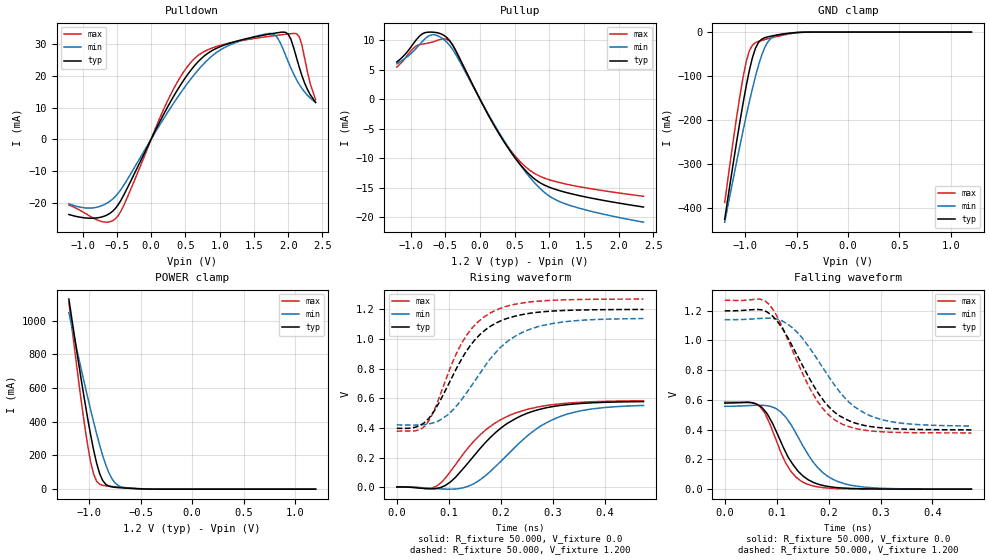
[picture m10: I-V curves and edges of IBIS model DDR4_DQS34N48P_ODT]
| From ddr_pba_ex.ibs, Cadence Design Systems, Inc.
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|   Model DDR4_DQS34N48P_ODT
[Model]   DDR4_DQS34N48P_ODT
Model_type I/O
Polarity   Non-Inverting
Enable   Active-High
Vinl =  0.823V
Vinh =  0.887V
C_comp   1.693pF   1.693pF   1.716pF
C_comp_pullup   0.525pF   0.576pF   0.518pF
C_comp_pulldown   1.168pF   1.117pF   1.198pF
[Model Spec]
Vinh   0.887V   NA   NA
Vinl   0.823V   NA   NA
Vmeas   0.840V   NA   NA
[Add Submodel]
|  Submodel_name   Mode
DDR4_DQS_ODT60   Non-Driving
[Temperature Range]   27.000   0.125k   -40.000
[Voltage Range]   1.200V   1.140V   1.270V
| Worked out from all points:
|   slope of the pulldown table from 0 to 0.18 V, typ, clamps not added: 23.3 ohm
|   slope of the pullup table from 0 to 0.18 V, typ, clamps not added: 45.9 ohm
|   GND clamp passes 1 mA (typ) near -0.50 V on its own axis
|   POWER clamp passes 1 mA (typ) near -0.46 V on its own axis
|   rising waveform, R_fixture 50.000, V_fixture 0.0: 20-80 % time 103ps typ, 110ps min, 100ps max; typ from 0.002 V to 0.578 V
|   rising waveform, R_fixture 50.000, V_fixture 1.200: 20-80 % time 83.6ps typ, 98.4ps min, 73ps max; typ from 0.397 V to 1.2 V
|   falling waveform, R_fixture 50.000, V_fixture 0.0: 20-80 % time 53.7ps typ, 63.6ps min, 45.1ps max; typ from 0.579 V to 0 V
|   falling waveform, R_fixture 50.000, V_fixture 1.200: 20-80 % time 81ps typ, 91.3ps min, 75.1ps max; typ from 1.2 V to 0.399 V
[Pulldown]
|Voltage   I(typ)   I(min)   I(max)
-1.2V     -23.72mA   -20.38mA   -20.68mA
-840mV    -24.88mA   -21.61mA   -24.88mA
-520mV    -21.78mA   -18mA      -25.05mA
400mV     16.1mA     13.66mA    18.67mA
640mV     23.35mA    20.64mA    25.58mA
960mV     28.73mA    27.44mA    29.28mA
1.76V     33.27mA    33.33mA    32.54mA
1.84V     33.56mA    32.14mA    32.76mA
2V        33.13mA    24.48mA    33.18mA
2.12V     25.82mA    18.86mA    33.28mA
2.2V      20.09mA    16.05mA    29.74mA
2.4V      11.64mA    11.56mA    12.48mA
[Pullup]
|Voltage   I(typ)   I(min)   I(max)
-1.2V     6.276mA    5.968mA    5.424mA
-960mV    9.395mA    8.108mA    8.597mA
-840mV    10.98mA    9.634mA    9.283mA
-720mV    11.33mA    10.8mA     9.54mA
-560mV    11.02mA    10.4mA     10.13mA
-400mV    9.244mA    8.51mA     9.292mA
280mV     -5.933mA   -5.721mA   -5.889mA
520mV     -10.14mA   -10.1mA    -9.786mA
760mV     -13.22mA   -13.77mA   -12.36mA
960mV     -14.69mA   -16.04mA   -13.47mA
1.2V      -15.64mA   -17.56mA   -14.24mA
2.36V     -18.24mA   -20.8mA    -16.42mA
[GND_clamp]
|Voltage   I(typ)   I(min)   I(max)
-1.2V     -426.2mA   -432.8mA   -388.3mA
-1.08V    -244.1mA   -290.9mA   -187.6mA
-1.02V    -160.2mA   -222.9mA   -101.2mA
-990mV    -121.8mA   -190.1mA   -66.76mA
-960mV    -87.12mA   -158.5mA   -42.47mA
-900mV    -36.37mA   -100.2mA   -23.99mA
-840mV    -16.17mA   -52.6mA    -18.98mA
-810mV    -12.75mA   -34.94mA   -17.06mA
-750mV    -9.219mA   -14.09mA   -13.42mA
-600mV    -3.476mA   -2.979mA   -5.372mA
-390mV    -77.95uA   -145.6uA   -88.64uA
1.2V      1.562nA    185.8nA    255.1pA
[POWER_clamp]
|Voltage   I(typ)   I(min)   I(max)
-1.2V     1.129A     1.047A     1.109A
-1.08V    651.1mA    713.3mA    524.8mA
-1.02V    430.1mA    553.1mA    270.8mA
-990mV    328mA      475.7mA    167mA
-960mV    234.7mA    400.6mA    90.32mA
-930mV    154.2mA    328.7mA    47.17mA
-900mV    91.53mA    260.8mA    29.3mA
-840mV    28.2mA     142.5mA    19.67mA
-780mV    13.3mA     60.49mA    15.94mA
-720mV    9.309mA    21.57mA    12.7mA
-660mV    6.902mA    8.818mA    9.642mA
1.2V      -4.11nA    -153.5nA   -871.8pA
[Ramp]
| variable   typ   min   max
dV/dt_r 0.348/0.105n   0.332/0.117n   0.351/0.105n
dV/dt_f 0.481/83.956p   0.430/97.879p   0.535/78.057p
R_load = 50.000
| The next line is not an IBIS keyword
| [Initial Delay]   0.325ns   0.500ns   0.200ns
[Rising Waveform]
R_fixture= 50.000
V_fixture= 0.0
V_fixture_min= 0.0
V_fixture_max= 0.0
|time   V(typ)   V(min)   V(max)
0s        1.711mV    1.158mV    451.4uV
65ps      -11.56mV   -7.321mV   -8.061mV
92ps      8.328mV    -12.86mV   55.58mV
148ps     209.5mV    22.65mV    308.6mV
190ps     368mV      139.1mV    434mV
226ps     457.4mV    264.3mV    497.4mV
268ps     518.5mV    391.6mV    538.6mV
318ps     553mV      481.4mV    563.8mV
378ps     569.8mV    529mV      576.8mV
475ps     577.5mV    551.4mV    583.4mV
[Rising Waveform]
R_fixture= 50.000
V_fixture= 1.200
V_fixture_min= 1.140
V_fixture_max= 1.270
|time   V(typ)   V(min)   V(max)
0s        397mV      420.5mV    378.1mV
55ps      441.7mV    423.1mV    415.2mV
66ps      484.5mV    429.8mV    472.7mV
89ps      620.6mV    465.5mV    673.9mV
125ps     865.5mV    591.9mV    972.8mV
155ps     1.012V     742.9mV    1.112V
185ps     1.096V     887.5mV    1.185V
227ps     1.154V     1.017V     1.234V
278ps     1.183V     1.089V     1.257V
475ps     1.2V       1.138V     1.27V
[Falling Waveform]
R_fixture= 50.000
V_fixture= 0.0
V_fixture_min= 0.0
V_fixture_max= 0.0
|time   V(typ)   V(min)   V(max)
0s        578.9mV    556.9mV    585.2mV
48ps      582.4mV    562.5mV    585.2mV
67ps      560.4mV    564.4mV    558.8mV
82ps      505.4mV    560.6mV    476.2mV
108ps     319mV      519.5mV    247.3mV
127ps     189mV      437.4mV    121.9mV
157ps     72.19mV    252.8mV    36.28mV
188ps     25.78mV    114mV      10.8mV
238ps     5.69mV     29.99mV    2.007mV
475ps     118uV      174.1uV    52.1uV
[Falling Waveform]
R_fixture= 50.000
V_fixture= 1.200
V_fixture_min= 1.140
V_fixture_max= 1.270
|time   V(typ)   V(min)   V(max)
0s        1.199V     1.139V     1.27V
67ps      1.207V     1.147V     1.278V
87ps      1.178V     1.15V      1.237V
111ps     1.081V     1.13V      1.088V
138ps     910.3mV    1.06V      870.8mV
177ps     662.7mV    880.3mV    599.1mV
217ps     503.1mV    673.4mV    453.9mV
248ps     448.4mV    558.4mV    411.2mV
298ps     413.5mV    471.5mV    386.5mV
475ps     398.7mV    424.4mV    378.1mV
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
